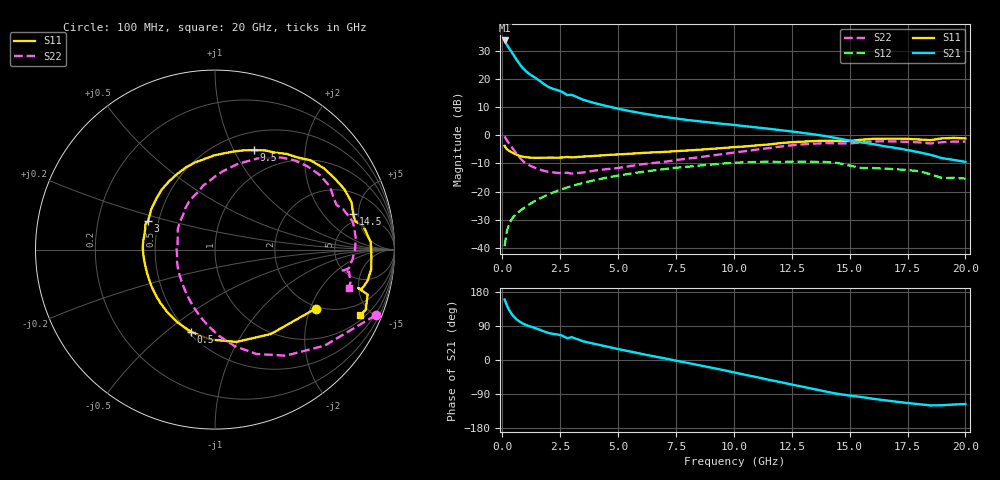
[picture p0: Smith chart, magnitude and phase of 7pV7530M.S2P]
! Infineon Technologies  Discrete & RF Semiconductors
! bfp620
! VCE = 0.75 V,  IC =  30 mA
! Common Emitter S-Parameters:  Sep 2002
# GHz  S  MA  R  50
!  f  S11  S21  S12  S22
! GHz  MAG  ANG  MAG  ANG  MAG  ANG  MAG  ANG
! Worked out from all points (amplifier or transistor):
!   59 points, 100 MHz to 20 GHz, reference 50 ohm
!   highest |S21| = 33.9 dB at 100 MHz (marker M1)
!   |S21| within 3 dB of that: start of sweep to 311.4 MHz
!   unconditionally stable (mu >= 1): 2.786 GHz to 2.822 GHz; 3.228 GHz to 10.15 GHz; 17.06 GHz to end of sweep
!   at 1 GHz: K = 0.78, MSG = 24.3 dB, |S12| = -25.5 dB
!   at 5.5 GHz: K = 1.04, MAG = 9.9 dB, |S12| = -13.7 dB
!   at 20 GHz: K = 1.46, MAG = -1.0 dB, |S12| = -15.4 dB
!   S11 on the Smith chart (normalised r, x): 100 MHz: 1.92, -2.18; 500 MHz: 0.52, -0.61; 3 GHz: 0.44, +0.17; 9.5 GHz: 0.70, +1.20; 14.5 GHz: 4.00, +4.30; 20 GHz: 1.25, -4.25
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0.1  0.6498 -30.4  49.43 159.5  0.0106 78.0  0.9673 -22.2
0.2  0.564 -56.5  41.29 143.7  0.0198 66.6  0.8123 -41.2
0.3  0.528 -76.9  35.57 131.3  0.0266 61.7  0.7103 -56.3
0.4  0.5019 -92.9  30.82 121.8  0.0318 58.7  0.6253 -68.4
0.5  0.4775 -106.2  26.64 114.3  0.036 56.7  0.5486 -78.5
0.6  0.4557 -117.5  23.01 108.3  0.0397 55.3  0.4811 -87.4
0.7  0.4384 -127.3  19.96 103.4  0.0431 54.5  0.425 -95.4
0.9  0.4168 -142.3  15.64 95.9  0.0498 53.9  0.3473 -109.1
1.1  0.4061 -152.6  13.12 90.7  0.0567 53.9  0.3038 -119.5
1.5  0.3987 -167.3  10.16 82.4  0.0709 53.1  0.2568 -136.6
2  0.4026 176.8  7.313 71.3  0.0889 50.5  0.2251 -158.9
2.8  0.4129 159.7  5.248 57.6  0.118 44.7  0.2158 175.9
3  0.4056 156.8  5.304 60.2  0.1254 43.1  0.209 174.4
3.5  0.4202 147.6  4.317 49.2  0.143 38.5  0.2187 161.9
5  0.4586 123.9  3.002 28.9  0.1926 23.8  0.2625 132.6
7  0.5086 96.4  2.142 4.5  0.2509 3.7  0.3381 105.4
9.5  0.5952 68.6  1.613 -26.0  0.3143 -23.5  0.4638 79.7
10.5  0.6372 57.9  1.461 -39.2  0.333 -36.2  0.524 69.9
13.5  0.7955 25.1  1.038 -77.2  0.3379 -71.6  0.7161 35.6
14.5  0.795 14.4  0.883 -89.5  0.3217 -86.8  0.7214 23.6
17  0.8769 -7.1  0.597 -109.9  0.2494 -102.6  0.7809 0.3
20  0.8852 -24.5  0.338 -116.1  0.1698 -113.5  0.776 -16.2
